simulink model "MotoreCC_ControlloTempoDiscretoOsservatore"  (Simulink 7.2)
settings: Solver=ode45  StartTime=0.0  StopTime=10.0  RelTol=1e-3
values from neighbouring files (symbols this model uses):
  A = [0   1   0    [Esercitazione06.m]
  B = [0  0   1]'    [Esercitazione06.m]
  C = [1  0   0]    [Esercitazione06.m]
  Kcontr = -acker(Az,Bz,[0.9 0 0])    [Esercitazione06.m]
  L = -acker(Az',Cz',[0 0 0])'    [Esercitazione06.m]
  Ts = 0.1    [Esercitazione06.m]
  X0 = [0.5 2 0.3]'    [Esercitazione06.m]
undefined symbols (not defined in the file or in its folder): Az, Bz, Cz
libraries: simulink x1

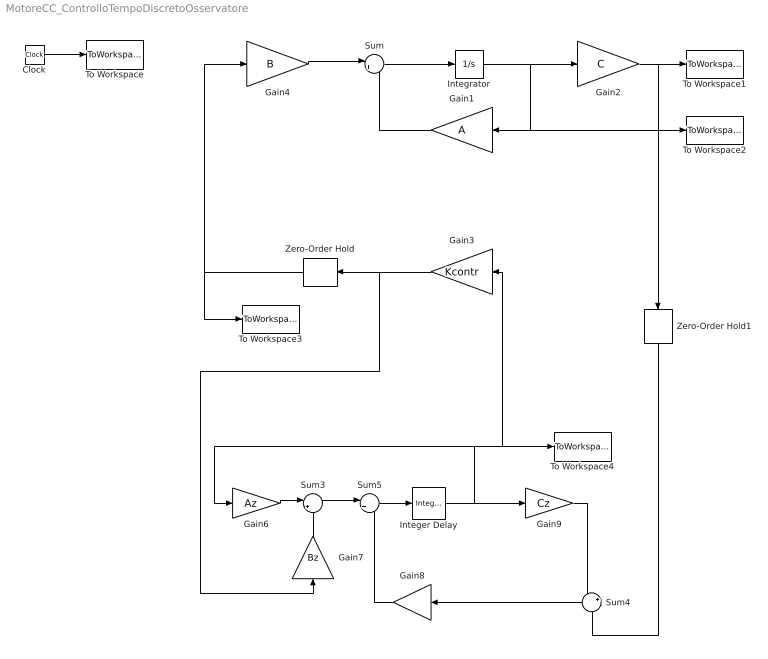
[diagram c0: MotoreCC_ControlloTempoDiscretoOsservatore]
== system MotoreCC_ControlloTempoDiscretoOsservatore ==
  Clock : Clock
  Gain1 : Gain  Orientation=left  Gain=A  Multiplication=Matrix(K*u)  ParameterDataType=sfix(16)  ParameterScaling=2^0  OutDataType=sfix(16)  OutScaling=2^0
  Gain2 : Gain  Gain=C  Multiplication=Matrix(K*u)  ParameterDataType=sfix(16)  ParameterScaling=2^0  OutDataType=sfix(16)  OutScaling=2^0
  Gain3 : Gain  Orientation=left  Gain=Kcontr  Multiplication=Matrix(K*u)  ParameterDataType=sfix(16)  ParameterScaling=2^0  OutDataType=sfix(16)  OutScaling=2^0
  Gain4 : Gain  Gain=B  Multiplication=Matrix(K*u)  ParameterDataType=sfix(16)  ParameterScaling=2^0  OutDataType=sfix(16)  OutScaling=2^0
  Gain6 : Gain  Gain=Az  Multiplication=Matrix(K*u)  ParameterDataType=sfix(16)  ParameterScaling=2^0  OutDataType=sfix(16)  OutScaling=2^0
  Gain7 : Gain  Orientation=up  Gain=Bz  Multiplication=Matrix(K*u)  ParameterDataType=sfix(16)  ParameterScaling=2^0  OutDataType=sfix(16)  OutScaling=2^0
  Gain8 : Gain  Orientation=left  Gain=L  Multiplication=Matrix(K*u)  ParameterDataType=sfix(16)  ParameterScaling=2^0  OutDataType=sfix(16)  OutScaling=2^0
  Gain9 : Gain  Gain=Cz  Multiplication=Matrix(K*u)  ParameterDataType=sfix(16)  ParameterScaling=2^0  OutDataType=sfix(16)  OutScaling=2^0
  Integer Delay : simulink/Discrete/Integer Delay  vinit=[0 0 0]'  samptime=Ts  NumDelays=1
  Integrator : Integrator  InitialCondition=X0
  Sum : Sum  Inputs=|++  OutDataType=sfix(16)  OutScaling=2^0
  Sum3 : Sum  Inputs=|++  OutDataType=sfix(16)  OutScaling=2^0
  Sum4 : Sum  Orientation=left  Inputs=+-  OutDataType=sfix(16)  OutScaling=2^0
  Sum5 : Sum  Inputs=|++  OutDataType=sfix(16)  OutScaling=2^0
  To Workspace : ToWorkspace  VariableName=time  SampleTime=-1  SaveFormat=Array
  To Workspace1 : ToWorkspace  VariableName=y  SampleTime=-1  SaveFormat=Array
  To Workspace2 : ToWorkspace  VariableName=X  SampleTime=-1  SaveFormat=Array
  To Workspace3 : ToWorkspace  VariableName=ud  SampleTime=-1  SaveFormat=Array
  To Workspace4 : ToWorkspace  VariableName=Xs  SampleTime=-1  SaveFormat=Array
  Zero-Order Hold : ZeroOrderHold  Orientation=left  SampleTime=Ts
  Zero-Order Hold1 : ZeroOrderHold  Orientation=down  SampleTime=Ts
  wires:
  Gain1/1 -> Sum/2
  Sum/1 -> Integrator/1
  Integrator/1 -> Gain2/1, Gain1/1, To Workspace2/1
  Gain2/1 -> To Workspace1/1, Zero-Order Hold1/1
  Gain4/1 -> Sum/1
  Gain3/1 -> Zero-Order Hold/1, Gain7/1
  Zero-Order Hold/1 -> Gain4/1, To Workspace3/1
  Clock/1 -> To Workspace/1
  Gain6/1 -> Sum3/1
  Integer Delay/1 -> Gain9/1, Gain6/1, Gain3/1, To Workspace4/1
  Gain7/1 -> Sum3/2
  Sum4/1 -> Gain8/1
  Gain9/1 -> Sum4/1
  Gain8/1 -> Sum5/2
  Sum3/1 -> Sum5/1
  Sum5/1 -> Integer Delay/1
  Zero-Order Hold1/1 -> Sum4/2
